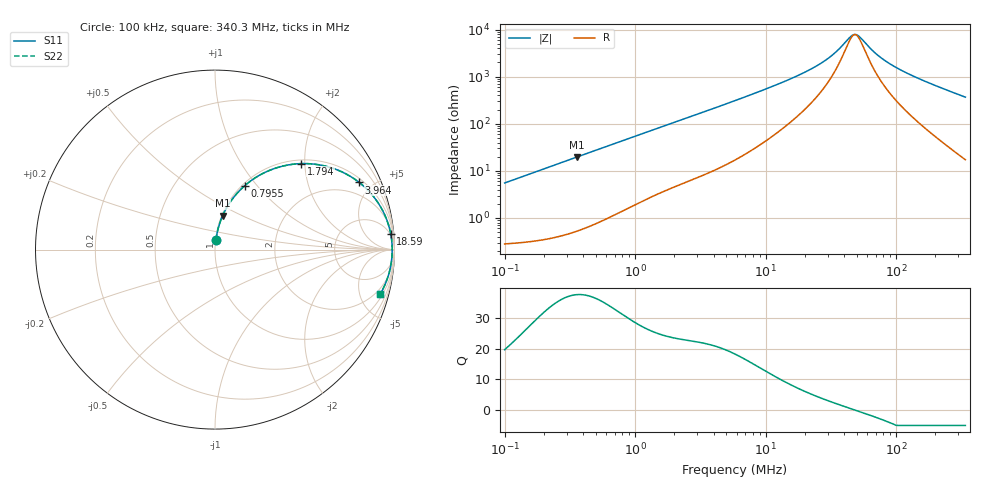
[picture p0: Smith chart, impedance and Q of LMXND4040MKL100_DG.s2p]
! LMXND4040MKL100_DG  S-PARAMETER MODEL  ( General Type )
! Model Generated by TAIYO YUDEN Corporation (https://www.yuden.co.jp/en/)
! Version 1.0
! TAIYO YUDEN Control No. 191023NI43SB-FBB
! Copyright(c) 2019 TAIYO YUDEN CO.,LTD. All Rights Reserved.
! Product Description (link to TY-COMPAS)
! https://ds.yuden.co.jp/TYCOMPAS/or/detail?pn=LMXND4040MKL100MDG&u=M
! Products Name : Inductors
! Characteristics :
!  Inductance : 10 uH , SRF(min) : 30 MHz , DC Resistance(max) : 0.204 Ohm
!  Rated Current : Saturation :800 mA , Temp Rise : 1100 mA (40 degC)
!  Case Size : 4.0 x 4.0 / 0.157 x 0.157 [mm/inch] , Thickness : 1.2 / 0.047 [mm/inch]
!  (Conditions: Temperature = 25 degC , DC Bias Current/Voltage = 0A / 0V)
! External Node Assignments :
!  1  o---GGG---o  2
! GND o---------o GND
! Frequency Range : 0.1MHz  -  340.31115MHz  [ 402 STEP ]
# MHz S RI R 50
! Freq[MHz].  S11 Real  S11 Imag  S21 Real  S21 Imag  S12 Real  S12 Imag  S22 Real  S22 Imag
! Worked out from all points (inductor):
!   401 points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, 100 kHz to 340.3 MHz, reference 50 ohm
!   read as one part in series: L = 8.77 uH near 104.2 kHz
!   highest Q = 37.5 at 360 kHz (marker M1), where L = 8.74 uH
!   self-resonance near 48.47 MHz
!   S11 on the Smith chart (normalised r, x): 100 kHz: 1.01, +0.11; 795.5 kHz: 1.03, +0.87; 1.794 MHz: 1.08, +1.92; 3.964 MHz: 1.20, +4.19; 18.59 MHz: 4, +22; 340.3 MHz: 1.34, -7.33
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0.1  0.00582 0.0547  0.9942 -0.0547  0.9942 -0.0547  0.00582 0.0547
0.199622  0.0152 0.1078  0.9848 -0.1078  0.9848 -0.1078  0.0152 0.1078
0.359973  0.0423 0.1883  0.9577 -0.1883  0.9577 -0.1883  0.0423 0.1883
0.390471  0.0489 0.2026  0.9511 -0.2026  0.9511 -0.2026  0.0489 0.2026
0.795478  0.1661 0.3564  0.8339 -0.3564  0.8339 -0.3564  0.1661 0.3564
1.524679  0.4056 0.4712  0.5944 -0.4712  0.5944 -0.4712  0.4056 0.4712
1.793974  0.4807 0.4791  0.5193 -0.4791  0.5193 -0.4791  0.4807 0.4791
2.586726  0.6475 0.4561  0.3525 -0.4561  0.3525 -0.4561  0.6475 0.4561
3.964368  0.8034 0.3743  0.1966 -0.3743  0.1966 -0.3743  0.8034 0.3743
5.953437  0.8963 0.2784  0.1037 -0.2784  0.1037 -0.2784  0.8963 0.2784
11.18119  0.9615 0.1538  0.0385 -0.1538  0.0385 -0.1538  0.9615 0.1538
18.5879  0.9796 0.0851  0.0204 -0.0851  0.0204 -0.0851  0.9796 0.0851
22.77862  0.983 0.0637  0.017 -0.0637  0.017 -0.0637  0.983 0.0637
31.53569  0.9861 0.0341  0.0139 -0.0341  0.0139 -0.0341  0.9861 0.0341
36.35886  0.9869 0.0225  0.0131 -0.0225  0.0131 -0.0225  0.9869 0.0225
44.5561  0.9874 0.0065  0.0126 -0.0065  0.0126 -0.0065  0.9874 0.0065
48.33101  0.9874 0.000211  0.0126 -0.000211  0.0126 -0.000211  0.9874 0.000211
52.42575  0.9874 -0.00607  0.0126 0.00607  0.0126 0.00607  0.9874 -0.00607
68.28584  0.9867 -0.027  0.0133 0.027  0.0133 0.027  0.9867 -0.027
88.94399  0.985 -0.0497  0.015 0.0497  0.015 0.0497  0.985 -0.0497
153.9991  0.9753 -0.1091  0.0247 0.1091  0.0247 0.1091  0.9753 -0.1091
340.3111  0.9208 -0.2476  0.0792 0.2476  0.0792 0.2476  0.9208 -0.2476
